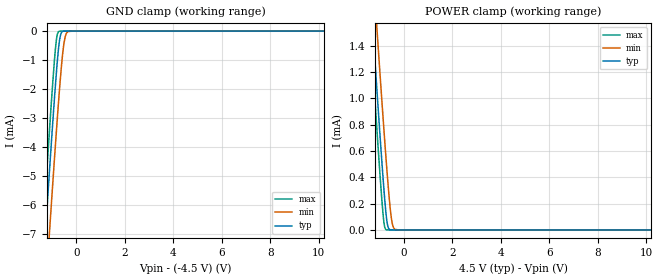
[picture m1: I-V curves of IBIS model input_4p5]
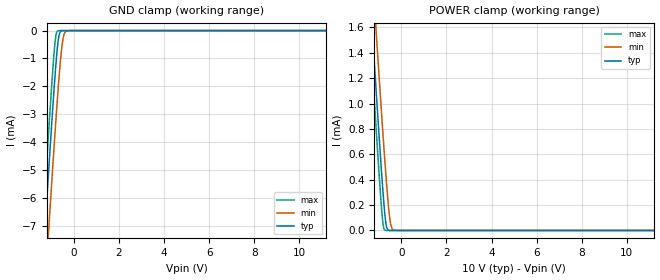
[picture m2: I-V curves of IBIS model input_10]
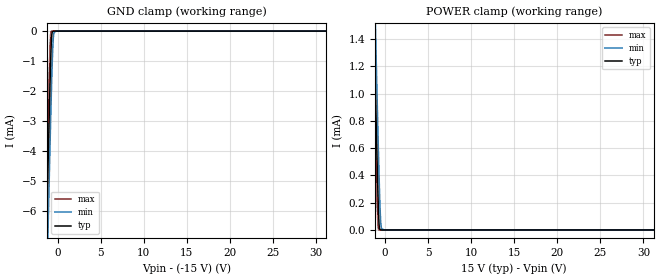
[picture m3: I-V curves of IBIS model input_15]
|Texas Instruments Incorporated
| MUX36xxx 36-V,Low-Capacitance,Low Charge Injection,Precision Analog
| Multiplexers
| Marketing part#   Digital Voltage Range   Package-type   #pins
| MUX36D08   4.5V-36.0V   TSSOP   28
[IBIS Ver]   4.1
[File name]   mux36d08.ibs
[File Rev]   2.0
[Date]   01/14/2016
[Source]
| Texas Instruments Incorporated.
| Analog-eLab Design Center, HPA
| 12500 TI Blvd
| Dallas, TX -75243
[Notes]   Revision History:
| Rev 2.0: 1/14/2016
| - Updated model with no leakage
| Rev 1.0: 12/09/2015
| - Relative part of MUX36S08.
| - Model generated from simulations in SPECTRE
| - Model matched to SPICE simulation
| - C_comp although listed in numerical order of value are
|   obtained from varying PVT conditions. For PVT conditions for
|   each specific value refer the buffer description under
|   respective [Model]. IBIS model user is responsible for using
|   appropriate C_comp to simulate for Signal Integrity.
[Disclaimer]
| This model is designed as an aid for customers of Texas Instruments.
| TI and its licensors and suppliers make no warranties, either expressed
| or implied, with respect to this  model, including the warranties of
| merchantability or fitness for a particular purpose. The model is
| provided solely on an "as is" basis. The entire risk as to its quality
| and performance is with the customer.
[Copyright]
(C) Copyright 2016 Texas Instruments Incorporated.All rights reserved.
|   MUX36D04PW
[Component]   MUX36D08
[Manufacturer]   TI
[Package]   |28 TSSOP - PW package
|   typ   min   max
R_pkg   0.115   0.063   0.148
L_pkg   2.909nH  2.079nH 4.166nH
C_pkg   0.519pF   0.426pF   0.680pF
[Pin]  signal_name   model_name   R_pin   L_pin   C_pin
1   VDD   POWER   NA   NA   NA
2   DB   NC   NA   NA   NA
3   NC   NC   NA   NA   NA
4   S8B   NC   NA   NA   NA
5   S7B   NC   NA   NA   NA
6   S6B   NC   NA   NA   NA
7   S5B   NC   NA   NA   NA
8   S4B   NC   NA   NA   NA
9   S3B   NC   NA   NA   NA
10   S2B   NC   NA   NA   NA
11   S1B   NC   NA   NA   NA
12   GND   GND   NA   NA   NA
13   NC   NC   NA   NA   NA
14   NC   NC   NA   NA   NA
15   A2   INPUT   NA   NA   NA
16   A1   INPUT   NA   NA   NA
17   A0   INPUT   NA   NA   NA
18   EN   INPUT   NA   NA   NA
19   S1A   NC   NA   NA   NA
20   S2A   NC   NA   NA   NA
21   S3A   NC   NA   NA   NA
22   S4A   NC   NA   NA   NA
23   S5A   NC   NA   NA   NA
24   S6A   NC   NA   NA   NA
25   A7A   NC   NA   NA   NA
26   A8A   NC   NA   NA   NA
27   VSS   GND   NA   NA   NA
28   DA   NC   NA   NA   NA
|   Model Selectors
[Model Selector] INPUT
input_4p5   4.5V  digital Input
input_10   10V   digital Input
input_15   15V   digital Input
input_36   36V   digital Input
| Models and submodels in the file (4): input_4p5 (Input), input_10 (Input), input_15 (Input), input_36 (Input)
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|   input_4p5 Model
[Model]   input_4p5
Model_type   Input
Vinl = 0.8
Vinh = 2.0
|   typ   min   max
|   (nom PVT)   (fast PVT)   (slow PVT)
C_comp   4.668e-13   4.656e-13   4.681e-13
| Where nom  PVT is Nominal Process, 9V, 27C
|   Fast PVT is Strong Process,  9.02V, -40C
|   Slow PVT is Weak Process,   8.98V, 125C
[Voltage Range]   9   8.98   9.02
|Junction Temperature
[Temperature Range]   27   125   -40
[Power Clamp Reference]   4.5   4.49   4.51
[GND Clamp Reference]   -4.5   -4.49   -4.51
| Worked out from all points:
|   GND clamp passes 1 mA (typ) near -0.78 V on its own axis
|   POWER clamp passes 1 mA (typ) near -1.08 V on its own axis
[GND Clamp]
|   Voltage   I(typ)   I(min)   I(max)
-9V       -110.9mA   -112.3mA   -110.2mA
-1.376V   -8.295mA   -10.41mA   -6.907mA
-1.314V   -7.492mA   -9.61mA    -6.097mA
-1.214V   -6.21mA    -8.334mA   -4.807mA
-1.143V   -5.295mA   -7.422mA   -3.889mA
-1.071V   -4.4mA     -6.526mA   -2.996mA
-836.9mV  -1.607mA   -3.651mA   -415.1uA
-702mV    -383.4uA   -2.114mA   -6.148uA
-630mV    -82.53uA   -1.375mA   -250.7nA
-513.9mV  -2.396uA   -451.9uA   0A
-342mV    0A         -16.72uA   0A
18V       0A         0A         0A
[POWER Clamp]
|   Voltage   I(typ)   I(min)   I(max)
-9V       24.14mA    24.27mA    24.22mA
-1.376V   1.814mA    2.273mA    1.524mA
-1.314V   1.639mA    2.1mA      1.345mA
-1.214V   1.359mA    1.824mA    1.061mA
-1.143V   1.159mA    1.626mA    858.5uA
-1.071V   963.1uA    1.432mA    661.3uA
-845.9mV  371uA      829.6uA    101.2uA
-711mV    87.38uA    489.9uA    1.013uA
-639mV    16.43uA    322.8uA    31.6nA
-513.9mV  226.1nA    91.1uA     0A
-360mV    0A         3.703uA    0A
18V       0A         0A         0A
|   input_10 Model
[Model]   input_10
Model_type   Input
Vinl = 0.8
Vinh = 2.0
|   typ   min   max
|   (nom PVT)   (fast PVT)   (slow PVT)
C_comp   4.758e-13   4.719e-13   4.784e-13
| Where nom  PVT is Nominal Process, 10V, 27C
|   Fast PVT is Strong Process,  10.1V, -40C
|   Slow PVT is Weak Process,   9.9V, 125C
[Voltage Range]   10   9.9   10.1
|Junction Temperature
[Temperature Range]   27   125   -40
[Power Clamp Reference]   10   9.9   10.1
[GND Clamp Reference]   0   0   0
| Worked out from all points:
|   GND clamp passes 1 mA (typ) near -0.78 V on its own axis
|   POWER clamp passes 1 mA (typ) near -1.09 V on its own axis
[GND Clamp]
|   Voltage   I(typ)   I(min)   I(max)
-10V      -124.4mA   -125.7mA   -123.8mA
-1.405V   -8.658mA   -10.77mA   -7.272mA
-1.29V    -7.169mA   -9.29mA    -5.771mA
-1.12V    -4.997mA   -7.125mA   -3.591mA
-852.4mV  -1.767mA   -3.824mA   -530.9uA
-770mV    -915.6uA   -2.861mA   -74.71uA
-697.9mV  -352.5uA   -2.06mA    -4.952uA
-634.6mV  -91.28uA   -1.411mA   -299.3nA
-525.7mV  -3.487uA   -517.9uA   0A
-446.5mV  -210.5nA   -154.9uA   0A
-344.4mV  0A         -17.35uA   0A
20V       0A         0A         0A
[POWER Clamp]
|   Voltage   I(typ)   I(min)   I(max)
-10V      27.09mA    27.17mA    27.21mA
-1.405V   1.893mA    2.351mA    1.604mA
-1.29V    1.568mA    2.031mA    1.274mA
-1.12V    1.094mA    1.562mA    792.7uA
-852.4mV  384.4uA    844.1uA    111.5uA
-798.9mV  257.7uA    706.2uA    31.95uA
-710mV    84.36uA    485.3uA    932.4nA
-644.5mV  18.81uA    332.9uA    39.9nA
-520mV    272.3nA    98.28uA    0A
-426.7mV  0A         17.74uA    0A
-364.6mV  0A         4.08uA     0A
20V       0A         0A         0A
|   input_15 Model
[Model]   input_15
Model_type   Input
Vinl = 0.8
Vinh = 2
|   typ   min   max
|   (nom PVT)   (fast PVT)   (slow PVT)
C_comp   4.413e-13   4.401e-13   4.413e-13
| Where nom  PVT is Nominal Process, 30V, 27C
|   Fast PVT is Strong Process,  30.2V, -40C
|   Slow PVT is Weak Process,   29.8V, 125C
[Voltage Range]   30   29.8   30.2
|Junction Temperature
[Temperature Range]   27   125   -40
[Power Clamp Reference]   15   14.9   15.1
[GND Clamp Reference]   -15   -14.9   -15.1
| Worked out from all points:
|   GND clamp passes 1 mA (typ) near -0.80 V on its own axis
|   POWER clamp passes 1 mA (typ) near -1.11 V on its own axis
[GND Clamp]
|   Voltage   I(typ)   I(min)   I(max)
-30V      -414.7mA   -439.3mA   -396.3mA
-1.431V   -8.735mA   -10.85mA   -7.348mA
-1.32V    -7.298mA   -9.42mA    -5.9mA
-1.243V   -6.308mA   -8.434mA   -4.903mA
-1.14V    -4.997mA   -7.127mA   -3.59mA
-1.08V    -4.245mA   -6.372mA   -2.841mA
-840mV    -1.415mA   -3.443mA   -298.2uA
-690mV    -207.7uA   -1.769mA   -1.813uA
-557.6mV  -5.645uA   -596.4uA   0A
-468.2mV  -250.5nA   -160.2uA   0A
-140.4mV  0A         -45.72nA   0A
60V       0A         0A         0A
[POWER Clamp]
|   Voltage   I(typ)   I(min)   I(max)
-30V      154.1mA    237.5mA    89.01mA
-1.431V   1.91mA     2.368mA    1.621mA
-1.303V   1.547mA    2.011mA    1.252mA
-1.213V   1.297mA    1.763mA    997.9uA
-1.08V    929.2uA    1.399mA    626.9uA
-917.4mV  497.5uA    962.3uA    207.2uA
-840mV    306.4uA    760.6uA    59.03uA
-706.6mV  55.02uA    429.7uA    308.9nA
-587.4mV  1.76uA     175.1uA    0A
-498mV    64.51nA    49.96uA    0A
-21.2mV   0A         0A         0A
60V       0A         0A         0A
